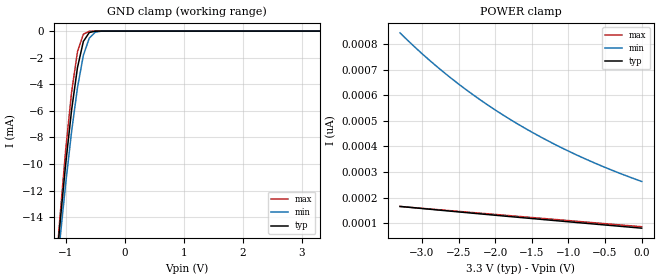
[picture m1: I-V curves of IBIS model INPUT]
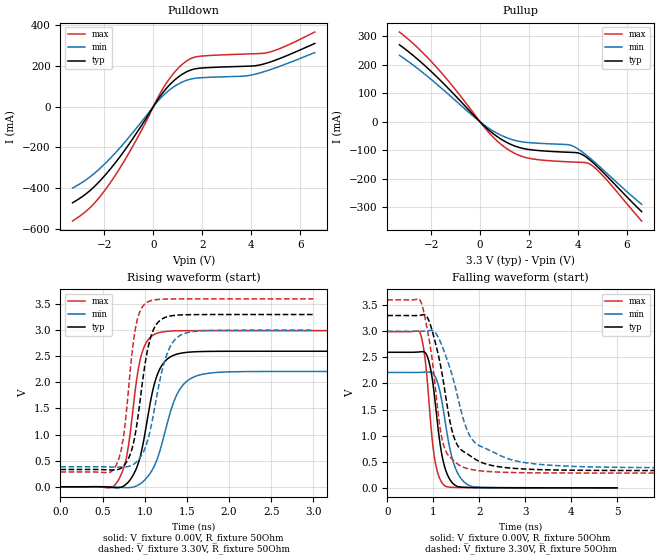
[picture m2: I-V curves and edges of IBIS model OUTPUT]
|   DIODES INCORPORATED
|   IBIS Model of PI49FCT3803
|   Product Family: 49FCT
|   TSSOP Package (L)
[IBIS Ver] 3.2
[Comment char] |_char
[File Name] pi49fct3803_l_33v.ibs
[File Rev] 1.0
[Source] File originated at Diodes Incorporated.
[Date] 06/20/18
[Disclaimer] (C) Copyright DIODES INCORPORATED
   All rights reserved
  Diodes Incorporated hereby grants the user of
  this IBIS model a non-exclusive, nontransferable license to
  use this IBIS model under the following terms.
  This IBIS model is provided on an "AS IS" basis and Diodes
  makes absolutely no warranty with respect to the information
  contained herein. DIODES DISCLAIMS AND CUSTOMER WAIVES ALL
  WARRANTIES, EXPRESSED OR IMPLIED, INCLUDING WARRANTIES OF
  MERCHANTABILITY OR FITNESS FOR A PARTICULAR PURPOSE. The
  entire risk as to quality and performance is with the customer.
  Accordingly, in no event shall the company be liable for any
  damages, whether in contract or tort, including any lost
  profits or other incidental, consequential, exemplary, or
  punitive damages arising out of the use or application of the
  IBIS model provided in this package. Further, Diodes reserves
  the right to make changes without notice to any product herein
  to improve reliability, function, or design. Diodes does not
  convey any license under patent rights or any other intellectual
  property rights, including those of third parties.
  The user is granted this license only to use the IBIS model
  and is not granted rights to sell, load, rent, lease or license
  the IBIS model in whole or in part, or in modified form to anyone
  other than user. User may modify the IBIS model to suit its specific
  application but rights to derivative works and such modifications
  shall belong to Diodes.
  Diodes is not obligated to provide maintenance or support
  for the licensed IBIS model.
  Contact Diodes at ATTN: APPLICATION ENGINEERING / IBIS MODELS
  1545 Barber Ln. Milpitas, CA 95035
[Component] PI49FCT3803
[Manufacturer] Diodes Incorporated.
[Package]
| Variable   typ   min   max
R_pkg   0.05665ohm   0.05334ohm   0.05997ohm
L_pkg   1.99150nH   1.82200nH   2.76100nH
C_pkg   0.20800pF   0.16300pF   0.25300pF
[Pin]  signal_name   model_name   R_pin   L_pin   C_pin
1   BUF_IN   INPUT   0.05997   2.76100nH   0.25300pF
2   GND   GND   0.05776   2.54800nH   0.22300pF
3   CLK0   OUTPUT   0.05555   2.33500nH   0.19300pF
4   VDD   POWER   0.05334   2.12200nH   0.16300pF
5   CLK1   OUTPUT   0.05334   2.12200nH   0.16300pF
6   GND   GND   0.05555   2.33500nH   0.19300pF
7   CLK2   OUTPUT   0.05776   2.54800nH   0.22300pF
8   VDD   POWER   0.05997   2.76100nH   0.25300pF
9   GND   GND   0.05997   2.76100nH   0.25300pF
10   CLK3   OUTPUT   0.05776   2.54800nH   0.22300pF
11   VDD   POWER   0.05555   2.33500nH   0.19300pF
12   CLK4   OUTPUT   0.05334   2.12200nH   0.16300pF
13   GND   GND   0.05334   2.12200nH   0.16300pF
14   CLK5   OUTPUT   0.05555   2.33500nH   0.19300pF
15   CLK6   OUTPUT   0.05776   2.54800nH   0.22300pF
16   VDD   POWER   0.05997   2.76100nH   0.25300pF
| Models and submodels in the file (2): INPUT (Input), OUTPUT (Output)
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|   Model INPUT
[Model] INPUT
Model_type Input
Vinl = 800mV
Vinh = 2.00V
| variable   typ   min   max
C_comp   4.135pF   4.130pF   4.140pF
[Voltage Range]   3.300V   3.000V   3.600V
[GND Clamp Reference]   0.000V   0.000V   0.000V
[POWER Clamp Reference]   3.300V   3.000V   3.600V
[Temperature Range]   25   85   -40
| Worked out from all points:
|   GND clamp passes 1 mA (typ) near -0.71 V on its own axis
[GND Clamp]
| Voltage   I(typ)   I(min)   I(max)
-3.3V     -154.9mA   -141.3mA   -174.8mA
-1.2V     -19.82mA   -20.56mA   -20.04mA
-1.1V     -14.69mA   -15.86mA   -14.19mA
-1V       -10.03mA   -11.5mA    -8.965mA
-900mV    -5.964mA   -7.581mA   -4.618mA
-800mV    -2.752mA   -4.259mA   -1.564mA
-700mV    -779.3uA   -1.822mA   -233.1uA
-600mV    -107.7uA   -530.3uA   -14.11uA
-500mV    -8.69uA    -91.37uA   -442.1nA
-400mV    -460.2nA   -7.074uA   -8.817nA
3.3V      80.78pA    295.4pA    79.2pA
[POWER Clamp]
| Voltage   I(typ)   I(min)   I(max)
-3.3V     165.7pA    844.1pA    165.6pA
-3V       157.6pA    763pA      158.4pA
-2.6V     146.9pA    666.4pA    148.8pA
-2.2V     136.5pA    581.4pA    139.2pA
-1.8V     126.1pA    506.5pA    129.6pA
-1.4V     115.9pA    440.5pA    120pA
-900mV    103.2pA    368.5pA    108pA
-500mV    93.21pA    318.3pA    98.4pA
0V        80.78pA    263.4pA    86.4pA
|   Model OUTPUT
[Model] OUTPUT
Model_type Output
Vref =  0.000V
Rref =  500ohms
Vmeas = 1.650V
| variable   typ   min   max
C_comp   6.678p   6.396p   6.926p
[Voltage Range]   3.300V   3.000V   3.600V
[Pullup Reference]   3.300V   3.000V   3.600V
[Pulldown Reference]   0.000V   0.000V   0.000V
[POWER Clamp Reference]   3.300V   3.000V   3.600V
[GND Clamp Reference]   0.000V   0.000V   0.000V
[Temperature Range]   25   85   -40
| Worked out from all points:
|   slope of the pulldown table from 0 to 0.495 V, typ, clamps not added: 5.87 ohm
|   slope of the pullup table from 0 to 0.495 V, typ, clamps not added: 12.8 ohm
|   falling waveform, V_fixture 0.00V, R_fixture 50Ohm: 20-80 % time 235ps typ, 292ps min, 192ps max; typ from 2.6 V to 0 V
|   rising waveform, V_fixture 0.00V, R_fixture 50Ohm: 20-80 % time 198ps typ, 256ps min, 154ps max; typ from 0 V to 2.6 V
|   falling waveform, V_fixture 3.30V, R_fixture 50Ohm: 20-80 % time 403ps typ, 574ps min, 299ps max; typ from 3.3 V to 0.331 V
|   rising waveform, V_fixture 3.30V, R_fixture 50Ohm: 20-80 % time 167ps typ, 212ps min, 133ps max; typ from 0.331 V to 3.3 V
[Pulldown]
| Voltage   I(typ)   I(min)   I(max)
-3.3V     -472.6mA   -400.2mA   -562.4mA
-2.5V     -403.4mA   -337mA     -486.5mA
-1.8V     -313mA     -259mA     -381.3mA
-800mV    -150.3mA   -121.6mA   -186.3mA
400mV     70.26mA    54.38mA    90.48mA
800mV     123.3mA    94.65mA    159.9mA
1.3V      167.7mA    127.1mA    219.5mA
1.6V      182.9mA    137.6mA    240.2mA
1.9V      189.2mA    142mA      248mA
3.8V      199mA      151.4mA    259.2mA
4.7V      216.7mA    178.7mA    267mA
6.6V      311mA      266.2mA    367.2mA
[Pullup]
| Voltage   I(typ)   I(min)   I(max)
-3.3V     270.7mA    234mA      315.5mA
-2.6V     223.2mA    190.4mA    264mA
-1.8V     160.4mA    134.4mA    193.5mA
0V        94.24pA    307.2pA    100.8pA
900mV     -62.92mA   -48.69mA   -81.85mA
1.4V      -84.03mA   -64.29mA   -109.7mA
1.9V      -95.52mA   -71.9mA    -125.7mA
3.7V      -106.8mA   -81.81mA   -140.3mA
4.1V      -111.5mA   -100.7mA   -141.7mA
4.5V      -134.6mA   -127.8mA   -148.8mA
5.1V      -183.1mA   -173.9mA   -196.5mA
6.6V      -314.8mA   -289.1mA   -347.7mA
[Falling Waveform]
V_fixture = 0.00V
V_fixture_min = 0.00V
V_fixture_max = 0.00V
R_fixture = 50Ohm
C_fixture = 0F
|   Time   V(typ)   V(min)   V(max)
0s        2.596V     2.209V     2.992V
725ps     2.605V     2.212V     2.939V
800ps     2.604V     2.215V     2.612V
875ps     2.509V     2.218V     2V
1.025ns   1.773V     2.155V     590.3mV
1.145ns   862.4mV    1.846V     170.7mV
1.25ns    397.3mV    1.324V     38.76mV
1.46ns    59.65mV    430.1mV    8.17mV
1.8ns     7.078mV    38.68mV    3.692mV
5ns       105.6uV    394.6uV    14.93uV
[Rising Waveform]
V_fixture = 0.00V
V_fixture_min = 0.00V
V_fixture_max = 0.00V
R_fixture = 50Ohm
C_fixture = 0F
|   Time   V(typ)   V(min)   V(max)
0s        0V         2.656uV    0V
675ps     -19.07mV   -6.313mV   96.27mV
780ps     51.84mV    -16.54mV   534.8mV
915ps     412.1mV    26.27mV    2.174V
1.005ns   1.047V     138.9mV    2.724V
1.125ns   2.032V     440.3mV    2.928V
1.23ns    2.386V     988.6mV    2.972V
1.38ns    2.54V      1.764V     2.987V
1.6ns     2.587V     2.115V     2.991V
4ns       2.596V     2.209V     2.992V
[Falling Waveform]
V_fixture = 3.30V
V_fixture_min = 3.00V
V_fixture_max = 3.60V
R_fixture = 50Ohm
C_fixture = 0F
|   Time   V(typ)   V(min)   V(max)
0s        3.3V       3V         3.6V
720ps     3.306V     2.999V     3.583V
920ps     3.167V     3.014V     2.788V
1.14ns    2.427V     2.826V     1.197V
1.22ns    2.039V     2.651V     828.7mV
1.44ns    998mV      2.066V     526.7mV
1.66ns    694.5mV    1.302V     393.3mV
1.95ns    530.1mV    835.3mV    333.9mV
3.1ns     355.9mV    470.7mV    288.3mV
10ns      330.8mV    382.9mV    283.3mV
[Rising Waveform]
V_fixture = 3.30V
V_fixture_min = 3.00V
V_fixture_max = 3.60V
R_fixture = 50Ohm
C_fixture = 0F
|   Time   V(typ)   V(min)   V(max)
0s        330.8mV    382.9mV    283.3mV
660ps     324.4mV    376.6mV    409mV
750ps     401.5mV    378.3mV    976mV
850ps     733mV      414.9mV    2.573V
920ps     1.347V     506.4mV    3.253V
1.015ns   2.465V     788.4mV    3.521V
1.105ns   3.018V     1.405V     3.578V
1.24ns    3.243V     2.431V     3.596V
1.4ns     3.29V      2.879V     3.599V
3ns       3.3V       3V         3.6V
[Ramp]
| variable   typ   min   max
dV/dt_r   1.55808V/196.67p   1.32516V/254.58p   1.79598V/152.87p
dV/dt_f   1.77984V/403.24p   1.56924V/572.65p   1.98966V/298.25p
R_load = 50
